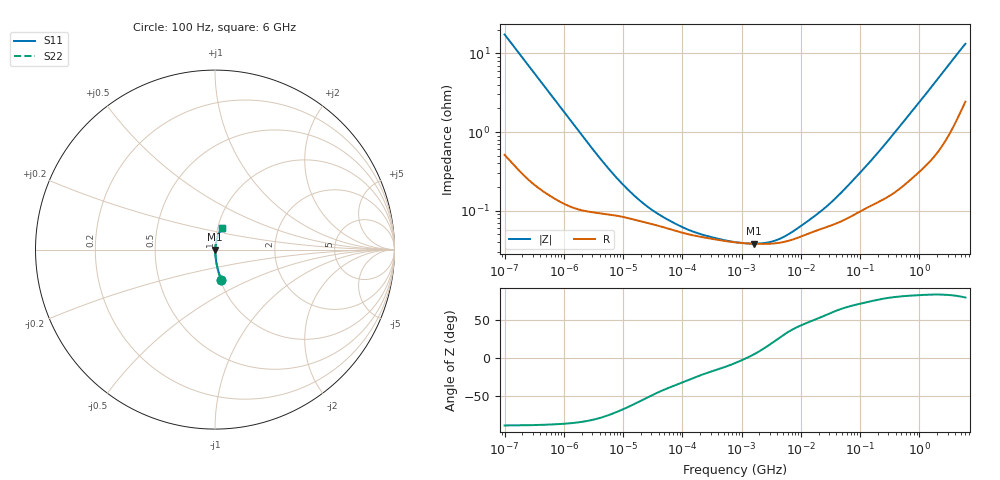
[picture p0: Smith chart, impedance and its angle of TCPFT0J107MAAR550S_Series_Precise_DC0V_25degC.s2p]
! TCPFT0J107MAAR550S Polymer Tantalum Capacitor Sparameter Model
! Model Generated by Samsung Electro-Mechanics
! Samsung Sparameter Version 5.0
! Date : Oct-21-2025
! Products : Polymer Tantalum Capacitor
! Characteristics :
!  Nominal Capacitance = 100uF
!  Capacitance Tolerance = +/-20%
!  ESR = 55 mohm max at 100kHz
!  Rated Voltage = 6.3Vdc
!  Size = 1206(unit:inch), 3216(unit:mm)
!  Length = 3.20+/-0.20mm
!  Width = 1.60+/-0.20mm
!  Thickness = 0.90+/-0.10mm
!  Lineup = Conductive Polymer Type
!  Feature = PFT
!  Measurement Temperature : 25degC.
!  DC bias Value = 0V
!  Frequency : 100Hz ~ 6GHz
! External Node Assignments :
!  1  o---||---o  2
# MHz S RI R 50.0
! Freq.  Real(S11)  Im(S11)  Real(S12)  Im(S12)  Real(S21)  Im(S21)  Real(S22)  Im(S22)
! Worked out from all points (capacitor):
!   300 points, 100 Hz to 6 GHz, reference 50 ohm
!   read as one part in series: C = 91.2 uF near 106.2 Hz
!   lowest |Z| = 38.2 mohm at 1.638 MHz (marker M1)
!   series resonance near 1.21 MHz, so ESL is about 190 pH
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0.0001  0.0339 -0.167  0.9661 0.167  0.9661 0.167  0.0339 -0.167
0.0001714451  0.0135 -0.1005  0.9865 0.1005  0.9865 0.1005  0.0135 -0.1005
0.0003313429  0.00491 -0.0531  0.9951 0.0531  0.9951 0.0531  0.00491 -0.0531
0.001998454  0.0011 -0.00909  0.9989 0.00909  0.9989 0.00909  0.0011 -0.00909
0.004907976  0.000924 -0.00379  0.9991 0.00379  0.9991 0.00379  0.000924 -0.00379
0.01007092  0.000835 -0.00196  0.9992 0.00196  0.9992 0.00196  0.000835 -0.00196
0.02066501  0.000729 -0.00106  0.9993 0.00106  0.9993 0.00106  0.000729 -0.00106
0.03993819  0.000641 -0.00063  0.9994 0.00063  0.9994 0.00063  0.000641 -0.00063
0.08700994  0.000541 -0.000361  0.9995 0.000361  0.9995 0.000361  0.000541 -0.000361
0.1583827  0.000483 -0.000232  0.9995 0.000232  0.9995 0.000232  0.000483 -0.000232
0.7981464  0.000395 -4.29e-05  0.9996 4.29e-05  0.9996 4.29e-05  0.000395 -4.29e-05
1.637756  0.00038 3.43e-05  0.9996 -3.43e-05  0.9996 -3.43e-05  0.00038 3.43e-05
2.807851  0.000379 0.00011  0.9996 -0.00011  0.9996 -0.00011  0.000379 0.00011
4.534038  0.000393 0.000205  0.9996 -0.000205  0.9996 -0.000205  0.000393 0.000205
7.321436  0.00043 0.000332  0.9996 -0.000332  0.9996 -0.000332  0.00043 0.000332
15.95059  0.000537 0.000622  0.9995 -0.000622  0.9995 -0.000622  0.000537 0.000622
29.03458  0.000631 0.000997  0.9994 -0.000997  0.9994 -0.000997  0.000631 0.000997
49.77836  0.000743 0.00158  0.9993 -0.00158  0.9993 -0.00158  0.000743 0.00158
137.8087  0.00112 0.0038  0.9989 -0.0038  0.9989 -0.0038  0.00112 0.0038
318.7652  0.00162 0.00812  0.9984 -0.00812  0.9984 -0.00812  0.00162 0.00812
1810.813  0.00663 0.0413  0.9934 -0.0413  0.9934 -0.0413  0.00663 0.0413
6000  0.0392 0.1218  0.9608 -0.1218  0.9608 -0.1218  0.0392 0.1218
